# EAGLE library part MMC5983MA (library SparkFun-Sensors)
High Performance 3-axis Magnetic Sensor The MMC5983MA is an AEC-Q100 qualified complete 3-axis magnetic sensor with on-chip signal processing and integrated I2C/SPI bus suitable for use in automotive applications. The device can be connected directly to a microprocessor, eliminating the need for A/D converters or timing resources. It can measure magnetic fields within the full scale range of ±8 Gauss (G), with 0.25mG/0.0625mG per LSB resolution at 16bits/18bits operation mode and 0.4 mG total RMS noise level, enabling heading accuracy of ±0.5° in electronic compass applications.
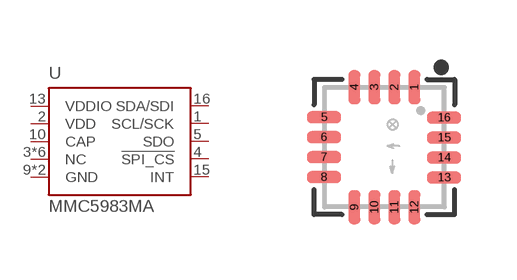
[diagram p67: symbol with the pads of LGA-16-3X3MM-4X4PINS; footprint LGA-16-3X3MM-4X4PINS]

Designator prefix U

## MMC5983MA_QFN16 (PROD_ID: IC-16314)  [LGA-16-3X3MM-4X4PINS]
1  SCL/SCK
2  VDD  pwr
3  NC  nc
4  !SPI_CS!  in
5  SDO  out
6  NC  nc
7  NC  nc
8  NC  nc
9  GND  pwr
10  CAP  pas
11  GND  pwr
12  NC  nc
13  VDDIO  pwr
14  NC  nc
15  INT  out
16  SDA/SDI

## Footprint LGA-16-3X3MM-4X4PINS (pad centres in mm)
3 x 3 mm 16 pin LGA package, pitch 0.5 mm.
smd 0.3 x 0.85: 1 0.754,1.498; 2 0.254,1.498; 3 -0.246,1.498; 4 -0.746,1.498; 9 -0.746,-1.506; 10 -0.246,-1.506; 11 0.254,-1.506; 12 0.754,-1.506
smd 0.85 x 0.3: 5 -1.508,0.746; 6 -1.508,0.246; 7 -1.508,-0.254; 8 -1.508,-0.754; 13 1.496,-0.764; 14 1.496,-0.264; 15 1.496,0.236; 16 1.496,0.736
